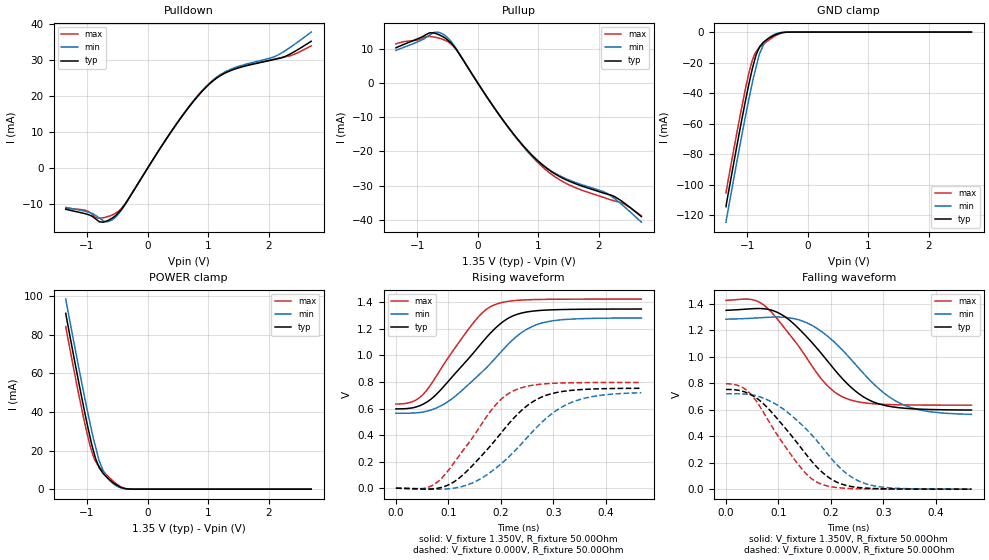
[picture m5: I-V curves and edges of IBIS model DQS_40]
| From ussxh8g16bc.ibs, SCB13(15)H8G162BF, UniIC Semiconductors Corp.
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| MODEL DQS_40 (40 Ohm Data Strobe I/O with no ODT, 800-2133Mbps)
[Model]   DQS_40
Model_type   I/O
Vinl = 545.000mV
Vinh = 805.000mV
Vmeas = 675.000mV
Vref = 675.000mV
Cref = 0.0pF
Rref = 25.000Ohm
|   typ   min   max
|C_comp   1.050pF   1.000pF   1.100pF
C_comp_pullup   0.5250pF   0.5000pF   0.5500pF
C_comp_pulldown   0.5250pF   0.5000pF   0.5500pF
[Model Spec]
| Input threshold voltage corners
Vinl   0.5450V   0.5115V   0.5825V
Vinh   0.8050V   0.7715V   0.8425V
| Measurement voltage corners
Vmeas   0.6750V   0.6415V   0.7125V
| Timing spec test load voltage corners
Vref   0.6750V   0.6415V   0.7125V
| Dynamic Overshoot Parameters from DDR3L Specification
|D_overshoot_ampl_h   0.40   NA   NA
|D_overshoot_ampl_l   0.40   NA   NA
|D_overshoot_area_h   0.11n   NA   NA
|D_overshoot_area_l   0.11n   NA   NA
[Receiver Thresholds]
|Vth   =  0.675V
|Vth_min  =  0.6615V
|Vth_max  =  0.6885V
|Vinh_ac  =  0.130V
|Vinh_dc  =  0.090V
|Vinl_ac  = -0.130V
|Vinl_dc  = -0.090V
|Tslew_ac =  5.000ns |Not specified, so set to high value
|Threshold_sensitivity = 0.50
|Reference_supply Pullup_ref
|NOTE: If using the IBISCHK 4.2.1 or older parser, Differential receiver
|threshold parameters must be commented out because the parser generates
|errors for multiple differential models.
Vcross_low   = 0.545V
Vcross_high  = 0.805V
Vdiff_ac   = 260mV
Vdiff_dc   = 180mV
Tdiffslew_ac = 10.000ns |Not specified, so set to high value
[Voltage Range]   1.3500V   1.2830V   1.4250V
[Pullup Reference]   1.3500V   1.2830V   1.4250V
| Junction Temperature (Ambient temp is 40C typ, 85C min, 0C max)
[Temperature Range]   45.0   90.0   0.0
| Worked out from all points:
|   slope of the pulldown table from 0 to 0.203 V, typ, clamps not added: 37.7 ohm
|   slope of the pullup table from 0 to 0.203 V, typ, clamps not added: 37.4 ohm
|   GND clamp passes 1 mA (typ) near -0.48 V on its own axis
|   POWER clamp passes 1 mA (typ) near -0.45 V on its own axis
|   falling waveform, V_fixture 1.350V, R_fixture 50.00Ohm: 20-80 % time 103ps typ, 109ps min, 89.3ps max; typ from 1.35 V to 0.597 V
|   rising waveform, V_fixture 1.350V, R_fixture 50.00Ohm: 20-80 % time 101ps typ, 111ps min, 83.6ps max; typ from 0.597 V to 1.35 V
|   rising waveform, V_fixture 0.000V, R_fixture 50.00Ohm: 20-80 % time 103ps typ, 114ps min, 87.6ps max; typ from 0 V to 0.753 V
|   falling waveform, V_fixture 0.000V, R_fixture 50.00Ohm: 20-80 % time 95.3ps typ, 103ps min, 80.9ps max; typ from 0.753 V to 0 V
[Pulldown]
|   Voltage   I(typ)   I(min)   I(max)
-1.35V    -11.4mA    -10.87mA   -11.07mA
-1.015V   -12.69mA   -12mA      -11.73mA
-795mV    -14.86mA   -13.8mA    -13.84mA
-665mV    -14.56mA   -14.83mA   -13.44mA
-560mV    -13.55mA   -14.01mA   -12.79mA
-385mV    -10.3mA    -10.43mA   -10.19mA
515mV     13.14mA    13.2mA     13.09mA
1.05V     23.74mA    23.96mA    23.77mA
1.445V    27.45mA    27.84mA    27.62mA
2.13V     30.22mA    31.11mA    30.32mA
2.365V    31.7mA     33.56mA    31.16mA
2.7V      35.1mA     37.65mA    33.84mA
[GND Clamp]
|   Voltage   I(typ)   I(min)   I(max)
-1.35V    -114.4mA   -124.6mA   -105.4mA
-1.245V   -90.61mA   -100.9mA   -81.76mA
-1.105V   -60.48mA   -70.85mA   -52.11mA
-1.015V   -42.18mA   -52.23mA   -34.38mA
-925mV    -25.46mA   -34.83mA   -19.55mA
-855mV    -15.06mA   -23.01mA   -12.93mA
-800mV    -9.934mA   -14.48mA   -10.24mA
-715mV    -6.057mA   -6.91mA    -7.343mA
-615mV    -3.335mA   -2.939mA   -4.374mA
-505mV    -1.269mA   -799.5uA   -1.753mA
-345mV    -47.71uA   -29.49uA   -72.66uA
2.7V      0A         0A         0A
[Pullup]
|   Voltage   I(typ)   I(min)   I(max)
-1.35V    10.26mA    9.507mA    11.43mA
-795mV    14.65mA    13.96mA    13.59mA
-665mV    14.28mA    14.87mA    13.21mA
-560mV    13.37mA    14.13mA    12.65mA
-350mV    9.722mA    9.924mA    9.627mA
535mV     -13.64mA   -13.74mA   -13.76mA
810mV     -19.51mA   -19.58mA   -19.81mA
1.085V    -24.19mA   -24.11mA   -24.79mA
1.495V    -28.59mA   -28.27mA   -29.67mA
2.13V     -32.45mA   -32.24mA   -33.76mA
2.42V     -35.1mA    -36.18mA   -35.42mA
2.7V      -39.05mA   -40.69mA   -38.83mA
[POWER Clamp]
|   Voltage   I(typ)   I(min)   I(max)
-1.35V    91.15mA    98.58mA    84.31mA
-1.105V   50.34mA    58.03mA    44.26mA
-1.015V   36.4mA     43.87mA    31.05mA
-920mV    22.95mA    29.85mA    19.3mA
-855mV    15.55mA    21.44mA    14.32mA
-800mV    11.29mA    14.78mA    11.73mA
-720mV    7.69mA     8.611mA    8.864mA
-665mV    5.934mA    5.934mA    7.065mA
-560mV    3.172mA    2.652mA    3.939mA
-430mV    798.9uA    593.6uA    1.032mA
-305mV    80.62uA    46.1uA     56.63uA
2.7V      0A         0A         0A
[Ramp]
R_load = 50.00Ohm
|   typ   min   max
dV/dt_r   451.595mV/103.216ps 431.697mV/114.150ps 477.678mV/87.545ps
dV/dt_f   451.543mV/102.727ps 431.065mV/108.923ps 474.575mV/89.346ps
[Falling Waveform]
V_fixture = 1.350V
V_fixture_min = 1.283V
V_fixture_max = 1.425V
R_fixture = 50.00Ohm
|   Time   V(typ)   V(min)   V(max)
0s        1.35V      1.283V     1.425V
60ps      1.364V     1.293V     1.418V
108ps     1.313V     1.298V     1.233V
166ps     1.097V     1.231V     917.5mV
196ps     954.9mV    1.147V     770.7mV
226ps     816.9mV    1.033V     689.7mV
276ps     666.9mV    815.7mV    646.5mV
334ps     613.2mV    644.3mV    636.6mV
382ps     602.2mV    588.7mV    634.7mV
468ps     597.4mV    564.6mV    634mV
[Rising Waveform]
V_fixture = 1.350V
V_fixture_min = 1.283V
V_fixture_max = 1.425V
R_fixture = 50.00Ohm
|   Time   V(typ)   V(min)   V(max)
0s        597.4mV    564.6mV    634mV
38ps      611.5mV    567.6mV    663.8mV
68ps      674.6mV    590.4mV    789.3mV
102ps     814.8mV    659.6mV    996.5mV
146ps     1.011V     809mV      1.237V
186ps     1.192V     963.7mV    1.378V
226ps     1.303V     1.129V     1.414V
276ps     1.34V      1.242V     1.422V
324ps     1.347V     1.272V     1.424V
468ps     1.35V      1.283V     1.425V
[Rising Waveform]
V_fixture = 0.000V
V_fixture_min = 0.000V
V_fixture_max = 0.000V
R_fixture = 50.00Ohm
|   Time   V(typ)   V(min)   V(max)
0s        -2.121uV   -29.43uV   -12.99uV
66ps      -6.977mV   -6.127mV   13.84mV
108ps     41.2mV     -1.192mV   176.4mV
148ps     179.2mV    43.53mV    391.5mV
188ps     355mV      143.3mV    617.6mV
228ps     541.5mV    286.2mV    740.5mV
276ps     683.3mV    488.5mV    783.4mV
332ps     736.1mV    641.8mV    794mV
382ps     748.2mV    695.1mV    795.9mV
468ps     752.7mV    719.5mV    796.1mV
[Falling Waveform]
V_fixture = 0.000V
V_fixture_min = 0.000V
V_fixture_max = 0.000V
R_fixture = 50.00Ohm
|   Time   V(typ)   V(min)   V(max)
0s        752.7mV    719.5mV    796.1mV
36ps      733.6mV    718.1mV    756.3mV
68ps      656.5mV    691.9mV    601.8mV
100ps     521.1mV    629.2mV    395.6mV
136ps     347.9mV    516.6mV    195mV
158ps     236.2mV    432.4mV    96.26mV
178ps     147.7mV    342.5mV    44.06mV
226ps     31.55mV    130.2mV    6.918mV
272ps     6.683mV    34.56mV    1.712mV
468ps     -2.121uV   -29.43uV   -12.99uV
